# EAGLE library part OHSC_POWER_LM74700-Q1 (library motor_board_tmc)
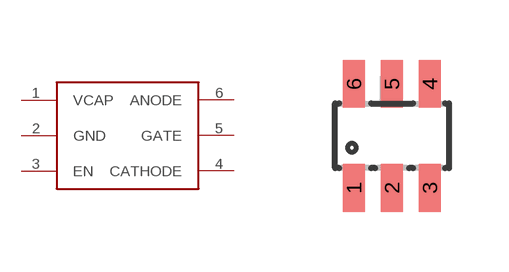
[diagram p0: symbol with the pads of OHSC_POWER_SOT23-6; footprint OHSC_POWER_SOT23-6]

Designator prefix U

## OHSC_POWER_LM74700-Q1  [OHSC_POWER_SOT23-6]
1  VCAP
2  GND
3  EN
4  CATHODE
5  GATE
6  ANODE

## Footprint OHSC_POWER_SOT23-6 (pad centres in mm)
smd 0.55 x 1.2: 1 -0.95,-1.3; 2 0,-1.3; 3 0.95,-1.3; 4 0.95,1.3; 5 0,1.3; 6 -0.95,1.3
